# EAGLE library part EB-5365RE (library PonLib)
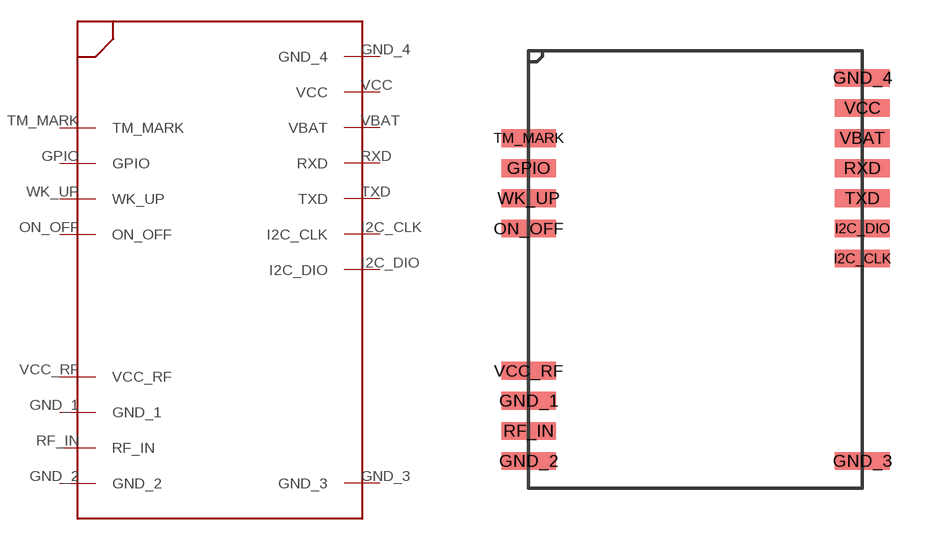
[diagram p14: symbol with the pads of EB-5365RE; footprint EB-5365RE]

Designator prefix -

## EB-5365RE  [EB-5365RE]
GND_1  GND_1
GND_2  GND_2
GND_3  GND_3
GND_4  GND_4
GPIO  GPIO
I2C_CLK  I2C_CLK
I2C_DIO  I2C_DIO
ON_OFF  ON_OFF
RF_IN  RF_IN
RXD  RXD
TM_MARK  TM_MARK
TXD  TXD
VBAT  VBAT
VCC  VCC
VCC_RF  VCC_RF
WK_UP  WK_UP

## Footprint EB-5365RE (pad centres in mm)
smd 2 x 0.65: GND_1 -6.1,-4.8; GND_2 -6.1,-7; GND_3 6.1,-7; GND_4 6.1,7; GPIO -6.1,3.7; I2C_CLK 6.1,0.4; I2C_DIO 6.1,1.5; ON_OFF -6.1,1.5; RF_IN -6.1,-5.9; RXD 6.1,3.7; TM_MARK -6.1,4.8; TXD 6.1,2.6; VBAT 6.1,4.8; VCC 6.1,5.9; VCC_RF -6.1,-3.7; WK_UP -6.1,2.6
